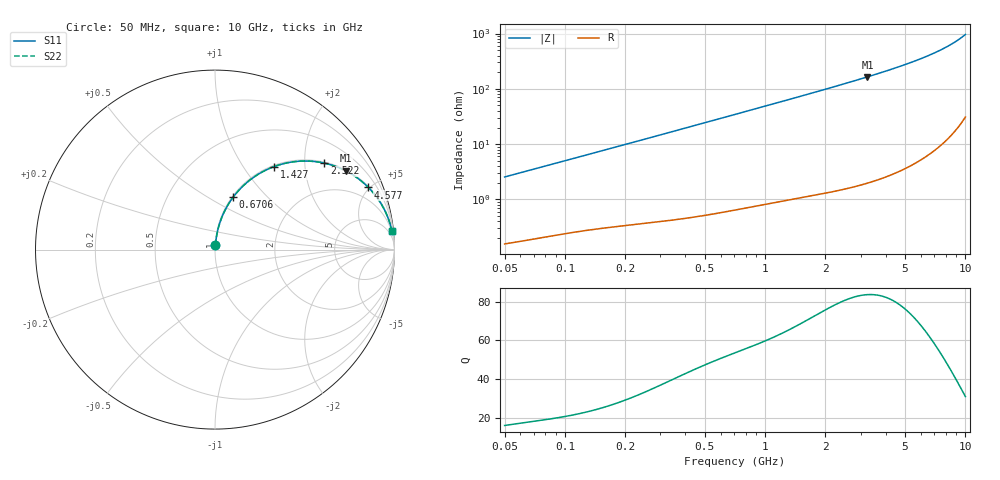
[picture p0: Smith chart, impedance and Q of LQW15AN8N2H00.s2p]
!Murata Part Number: LQW15AN8N2H00
!These Parameters are Measured in Series Mode Connection
!  o--[Z]--o
!Port1  Port2
!  o-------o
!Freq. Start=50[MHz] Stop=10[GHz], 401[Steps]
# Hz S RI R 50
!Freq.(Hz)	S 11(Real)	S 11(Imag)	S 21(Real)	S 21(Imag)	S 12(Real)	S 12(Imag)	S 22(Real)	S 22(Imag)
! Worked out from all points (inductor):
!   401 points, 50 MHz to 10 GHz, reference 50 ohm
!   read as one part in series: L = 8.06 nH near 51.34 MHz
!   highest Q = 83.6 at 3.244 GHz (marker M1), where L = 8.08 nH
!   S11 on the Smith chart (normalised r, x): 50 MHz: 1.00, +0.05; 670.6 MHz: 1.01, +0.65; 1.427 GHz: 1.02, +1.39; 2.522 GHz: 1.03, +2.51; 4.577 GHz: 1.06, +4.92; 10 GHz: 2, +19
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5e7  0.00221 0.0253  0.9978 -0.0253  0.9978 -0.0253  0.00221 0.0253
1.214486e8  0.00629 0.0599  0.9937 -0.0599  0.9937 -0.0599  0.00629 0.0599
1.956524e8  0.0125 0.0949  0.9875 -0.0949  0.9875 -0.0949  0.0125 0.0949
2.949953e8  0.0242 0.1405  0.9758 -0.1405  0.9758 -0.1405  0.0242 0.1405
4.628099e8  0.0528 0.213  0.9472 -0.213  0.9472 -0.213  0.0528 0.213
6.706172e8  0.101 0.292  0.899 -0.292  0.899 -0.292  0.101 0.292
7.071068e8  0.1106 0.3044  0.8894 -0.3044  0.8894 -0.3044  0.1106 0.3044
8.511793e8  0.151 0.3493  0.849 -0.3493  0.849 -0.3493  0.151 0.3493
1.011124e9  0.1991 0.3911  0.8009 -0.3911  0.8009 -0.3911  0.1991 0.3911
1.201124e9  0.2584 0.43  0.7416 -0.43  0.7416 -0.43  0.2584 0.43
1.426828e9  0.3289 0.4625  0.6711 -0.4625  0.6711 -0.4625  0.3289 0.4625
1.717543e9  0.4154 0.4859  0.5846 -0.4859  0.5846 -0.4859  0.4154 0.4859
2.095058e9  0.5156 0.4933  0.4844 -0.4933  0.4844 -0.4933  0.5156 0.4933
2.521925e9  0.61 0.4816  0.39 -0.4816  0.39 -0.4816  0.61 0.4816
3.243629e9  0.7282 0.4389  0.2718 -0.4389  0.2718 -0.4389  0.7282 0.4389
4.171863e9  0.8254 0.3736  0.1746 -0.3736  0.1746 -0.3736  0.8254 0.3736
4.577181e9  0.8548 0.346  0.1452 -0.346  0.1452 -0.346  0.8548 0.346
5.809576e9  0.9153 0.2713  0.0847 -0.2713  0.0847 -0.2713  0.9153 0.2713
7.181012e9  0.9525 0.204  0.0475 -0.204  0.0475 -0.204  0.9525 0.204
8.418147e9  0.9719 0.1545  0.0281 -0.1545  0.0281 -0.1545  0.9719 0.1545
9.738562e9  0.9843 0.1101  0.0157 -0.1101  0.0157 -0.1101  0.9843 0.1101
1e10  0.9861 0.1021  0.0139 -0.1021  0.0139 -0.1021  0.9861 0.1021
